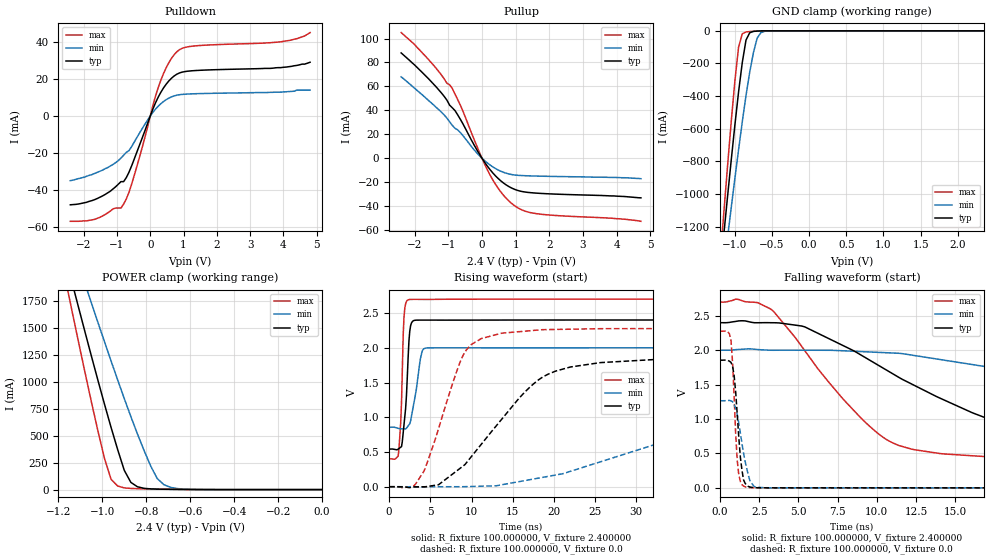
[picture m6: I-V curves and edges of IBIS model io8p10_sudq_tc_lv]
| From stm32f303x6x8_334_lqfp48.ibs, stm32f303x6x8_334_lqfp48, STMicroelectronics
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|   Model io8p10_sudq_tc_lv
[Model]  io8p10_sudq_tc_lv
Model_type I/O
Polarity   Non-Inverting
Enable   Active-Low
Vinl =   0.720000V
Vinh =   1.680000V
Vmeas =  1.200000V
Cref =   50.000000pF
Rref =   100.000000M
Vref =   0.0V
C_comp   1.378000pF   1.292700pF   1.486400pF
[Temperature Range]   25.000000   0.125000k   -40.000000
[Pullup Reference]   2.400000V   2.000000V   2.700000V
[Pulldown Reference]   0.0V   0.0V   0.0V
[POWER Clamp Reference]   2.400000V   2.000000V   2.700000V
[GND Clamp Reference]   0.0V   0.0V   0.0V
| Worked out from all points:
|   slope of the pulldown table from 0 to 0.36 V, typ, clamps not added: 25.7 ohm
|   slope of the pullup table from 0 to 0.36 V, typ, clamps not added: 26.8 ohm
|   GND clamp passes 1 mA (typ) near -0.67 V on its own axis
|   POWER clamp passes 1 mA (typ) near -0.60 V on its own axis
|   rising waveform, R_fixture 100.000000, V_fixture 2.400000: 20-80 % time 554ps typ, 889ps min, 361ps max; typ from 0.542 V to 2.4 V
|   rising waveform, R_fixture 100.000000, V_fixture 0.0: 20-80 % time 8.02ns typ, 22.7ns min, 3.78ns max; typ from 0 V to 1.85 V
|   falling waveform, R_fixture 100.000000, V_fixture 2.400000: 20-80 % time 10.1ns typ, 24ns min, 5.12ns max; typ from 2.4 V to 0.542 V
|   falling waveform, R_fixture 100.000000, V_fixture 0.0: 20-80 % time 377ps typ, 594ps min, 284ps max; typ from 1.85 V to 0 V
[Pulldown]
|Voltage   I(typ)   I(min)   I(max)
-2.4V     -47.8mA    -34.8mA    -56.7mA
-1.68V    -45.1mA    -31mA      -55.7mA
-1.12V    -39.3mA    -26.1mA    -50.05mA
-800mV    -35.33mA   -21.13mA   -47.42mA
-640mV    -30.33mA   -18.65mA   -41.16mA
-480mV    -23.12mA   -14mA      -31.94mA
240mV     10.22mA    5.339mA    15.38mA
480mV     17.22mA    8.864mA    26.1mA
800mV     22.59mA    11.27mA    34.68mA
1.36V     24.54mA    12.05mA    37.84mA
3.92V     26.1mA     12.9mA     40mA
4.8V      29mA       14mA       45mA
[Pullup]
|Voltage   I(typ)   I(min)   I(max)
-2.4V     88mA       68mA       105mA
-2V       77.9mA     58.5mA     95mA
-1.36V    59.6mA     42.5mA     75.1mA
-880mV    42.12mA    27.44mA    58.22mA
-560mV    28.45mA    18.75mA    39mA
-160mV    7.44mA     4.66mA     10.64mA
160mV     -6.607mA   -3.947mA   -9.704mA
480mV     -16.91mA   -9.806mA   -25.1mA
880mV     -24.9mA    -13.63mA   -37.75mA
1.2V      -27.87mA   -14.5mA    -43.37mA
1.6V      -29.13mA   -14.89mA   -46.24mA
4.72V     -33.1mA    -17.1mA    -52.7mA
[GND_clamp]
|Voltage   I(typ)   I(min)   I(max)
-2.4V     -7.358A    -6.372A    -8.78A
-1.2V     -1.489A    -1.65A     -1.416A
-1.15V    -1.254A    -1.461A    -1.124A
-1.1V     -1.024A    -1.273A    -838.2mA
-1.05V    -797.6mA   -1.088A    -563.1mA
-950mV    -374.6mA   -728.7mA   -100.8mA
-900mV    -194.3mA   -557.9mA   -18.01mA
-850mV    -56.94mA   -397.4mA   -7.08mA
-750mV    -3.582mA   -133.8mA   -2.771mA
-700mV    -1.516mA   -44.7mA    -1.516mA
-600mV    -235.4uA   -2.939mA   -209.5uA
2.35V     0A         0A         0A
[POWER_clamp]
|Voltage   I(typ)   I(min)   I(max)
-2.4V     9.979A     9.967A     9.901A
-1.17V    2.182A     2.481A     1.978A
-1.14V    1.945A     2.294A     1.683A
-1.11V    1.71A      2.108A     1.391A
-1.08V    1.476A     1.923A     1.102A
-1.05V    1.245A     1.739A     819.9mA
-960mV    578.2mA    1.196A     96.06mA
-900mV    179.5mA    846.7mA    16.04mA
-870mV    67.18mA    678.8mA    10.82mA
-780mV    6.749mA    219.9mA    5.853mA
-720mV    3.355mA    46.34mA    3.808mA
0V        0A         0A         0A
[Ramp]
| variable   typ   min   max
dV/dt_r  1.11324/8.00773n   0.75792/22.72286n   1.36566/3.77053n
dV/dt_f  1.11486/10.04030n   0.68695/24.01936n   1.37969/5.11177n
R_load = 100.000000
[Rising Waveform]
R_fixture= 100.000000
V_fixture= 2.400000
V_fixture_min= 2.000000
V_fixture_max= 2.700000
|time   V(typ)   V(min)   V(max)
0s        541.6mV    855mV      400.5mV
1.101ns   542.2mV    840.3mV    442.5mV
1.401ns   568.7mV    834mV      922.1mV
1.802ns   891.6mV    831.7mV    2.442V
2.102ns   1.317V     842.8mV    2.667V
2.302ns   1.856V     874.6mV    2.689V
2.703ns   2.355V     1.01V      2.696V
3.804ns   2.398V     1.846V     2.696V
4.404ns   2.398V     1.994V     2.696V
49.85ns   2.4V       2V         2.7V
[Rising Waveform]
R_fixture= 100.000000
V_fixture= 0.0
V_fixture_min= 0.0
V_fixture_max= 0.0
|time   V(typ)   V(min)   V(max)
0s        804.5pV    13.47nV    619.4pV
3.203ns   -1.631mV   -3.235mV   38.77mV
4.404ns   -401.8uV   -5.331mV   271.5mV
9.009ns   300.4mV    200.6uV    1.898V
13.61ns   963.6mV    26.7mV     2.208V
18.82ns   1.59V      138.3mV    2.261V
25.63ns   1.786V     357.3mV    2.275V
42.84ns   1.849V     950mV      2.276V
54.85ns   1.855V     1.159V     2.276V
99.7ns    1.855V     1.266V     2.276V
[Falling Waveform]
R_fixture= 100.000000
V_fixture= 2.400000
V_fixture_min= 2.000000
V_fixture_max= 2.700000
|time   V(typ)   V(min)   V(max)
0s        2.4V       2V         2.7V
3.203ns   2.4V       2V         2.602V
5.405ns   2.339V     2V         1.994V
10.01ns   1.793V     1.97V      802mV
14.21ns   1.284V     1.858V     493.7mV
20.22ns   787.8mV    1.645V     430.2mV
26.83ns   621.9mV    1.414V     407.1mV
37.04ns   566.4mV    1.142V     400.5mV
53.25ns   545mV      941.7mV    400.5mV
99.7ns    541.6mV    855mV      400.5mV
[Falling Waveform]
R_fixture= 100.000000
V_fixture= 0.0
V_fixture_min= 0.0
V_fixture_max= 0.0
|time   V(typ)   V(min)   V(max)
0s        1.855V     1.266V     2.276V
700.7ps   1.823V     1.265V     2.142V
900.9ps   1.633V     1.209V     1.33V
1.101ns   1.065V     1.064V     396.7mV
1.201ns   724.9mV    936.6mV    184.4mV
1.401ns   256mV      644.9mV    47.63mV
1.702ns   36.52mV    286.2mV    8.172mV
2.202ns   3.544mV    15.4mV     1.374mV
2.903ns   655uV      2.309mV    1.058mV
49.85ns   804.5pV    13.47nV    619.4pV
